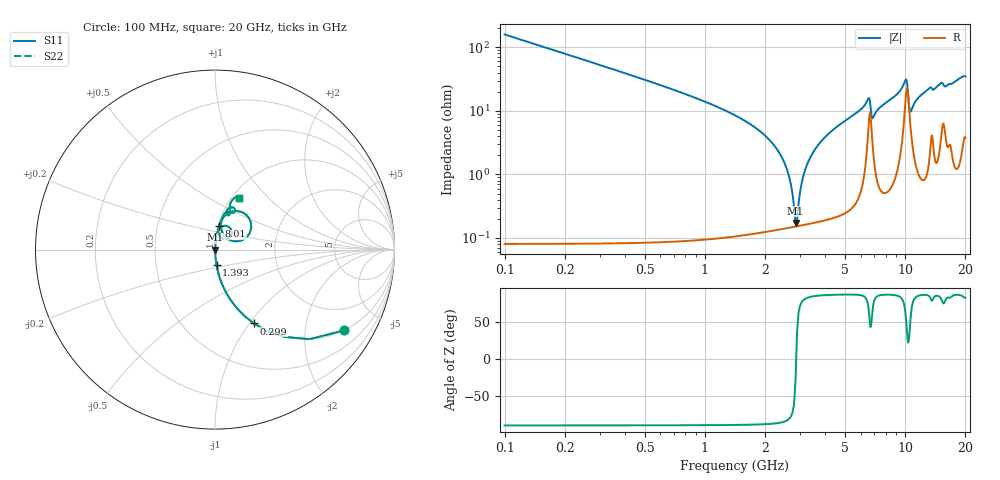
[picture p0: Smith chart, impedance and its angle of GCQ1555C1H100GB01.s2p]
!Murata Part Number: GCQ1555C1H100GB01
!These Parameters are Measured in Series Mode Connection
!Data Generated on Mar 13, 2026
!  o--ll--o
!Port1  Port2
!  o------o
!Operation Temp=25[degC], DC Bias Voltage=0[V]
!Freq. Start=100[MHz] Stop=20[GHz] 401[Steps]
# Hz S RI R 50
!Freq.(Hz) S11(Real) S11(Imag) S21(Real) S21(Imag) S12(Real) S12(Imag) S22(Real) S22(Imag)
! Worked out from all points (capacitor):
!   401 points, 100 MHz to 20 GHz, reference 50 ohm
!   read as one part in series: C = 10 pF near 199.5 MHz
!   lowest |Z| = 172 mohm at 2.836 GHz (marker M1)
!   series resonance near 2.857 GHz, so ESL is about 310 pH
!   S11 on the Smith chart (normalised r, x): 100 MHz: 1.00, -3.18; 299 MHz: 1.00, -1.05; 1.393 GHz: 1.00, -0.17; 8.01 GHz: 1.01, +0.27; 20 GHz: 1.08, +0.69
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1e8  0.7164 -0.4505  0.2836 0.4505  0.2836 0.4505  0.7164 -0.4505
2.99e8  0.2174 -0.4117  0.7826 0.4117  0.7826 0.4117  0.2174 -0.4117
5.975e8  0.0616 -0.2388  0.9384 0.2388  0.9384 0.2388  0.0616 -0.2388
1.3935e9  0.00856 -0.0863  0.9914 0.0863  0.9914 0.0863  0.00856 -0.0863
2.3885e9  0.00177 -0.0201  0.9982 0.0201  0.9982 0.0201  0.00177 -0.0201
2.5875e9  0.00155 -0.0111  0.9984 0.0111  0.9984 0.0111  0.00155 -0.0111
2.83625e9  0.00151 -0.00082  0.9985 0.00082  0.9985 0.00082  0.00151 -0.00082
2.93575e9  0.00155 0.00304  0.9984 -0.00304  0.9984 -0.00304  0.00155 0.00304
3.13475e9  0.00171 0.0104  0.9983 -0.0104  0.9983 -0.0104  0.00171 0.0104
3.43325e9  0.00213 0.0208  0.9979 -0.0208  0.9979 -0.0208  0.00213 0.0208
4.279e9  0.00426 0.0473  0.9957 -0.0473  0.9957 -0.0473  0.00426 0.0473
6.51775e9  0.0562 0.133  0.9438 -0.133  0.9438 -0.133  0.0562 0.133
6.7665e9  0.0631 0.0584  0.9369 -0.0584  0.9369 -0.0584  0.0631 0.0584
6.91575e9  0.0284 0.0706  0.9716 -0.0706  0.9716 -0.0706  0.0284 0.0706
8.01025e9  0.0224 0.1302  0.9776 -0.1302  0.9776 -0.1302  0.0224 0.1302
9.453e9  0.0585 0.1917  0.9415 -0.1917  0.9415 -0.1917  0.0585 0.1917
1.005e10  0.1736 0.1939  0.8264 -0.1939  0.8264 -0.1939  0.1736 0.1939
1.0647e10  0.0573 0.072  0.9427 -0.072  0.9427 -0.072  0.0573 0.072
1.159225e10  0.0341 0.1512  0.9659 -0.1512  0.9659 -0.1512  0.0341 0.1512
1.338325e10  0.0739 0.2095  0.9261 -0.2095  0.9261 -0.2095  0.0739 0.2095
1.67165e10  0.0882 0.233  0.9118 -0.233  0.9118 -0.233  0.0882 0.233
2e10  0.1331 0.2896  0.8669 -0.2896  0.8669 -0.2896  0.1331 0.2896
